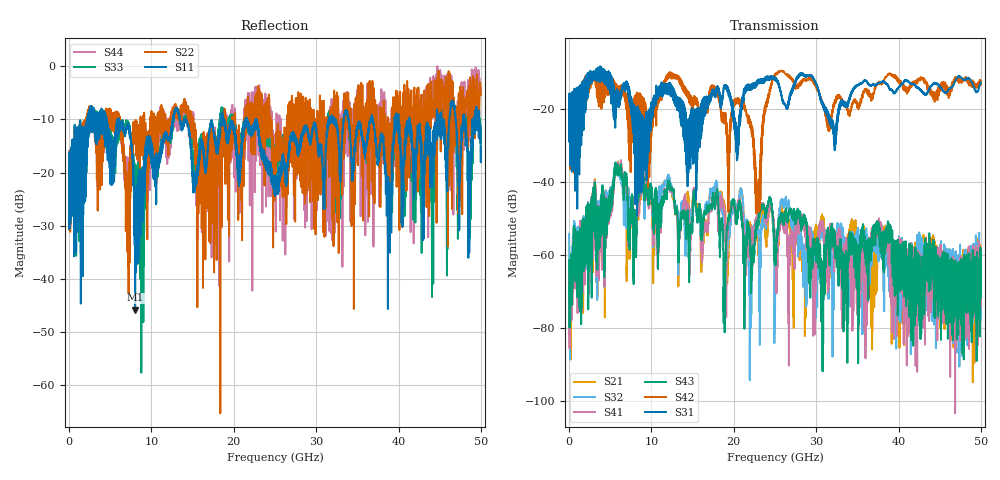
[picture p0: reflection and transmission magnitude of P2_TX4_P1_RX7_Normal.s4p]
!Keysight Technologies,N5225B,MY57041031,A.13.20.10
!Date: Friday, May 31, 2019 11:25:08
!Correction: S11(Full 4 Port(1,2,3,4))
!S12(Full 4 Port(1,2,3,4))
!S13(Full 4 Port(1,2,3,4))
!S14(Full 4 Port(1,2,3,4))
!S21(Full 4 Port(1,2,3,4))
!S22(Full 4 Port(1,2,3,4))
!S23(Full 4 Port(1,2,3,4))
!S24(Full 4 Port(1,2,3,4))
!S31(Full 4 Port(1,2,3,4))
!S32(Full 4 Port(1,2,3,4))
!S33(Full 4 Port(1,2,3,4))
!S34(Full 4 Port(1,2,3,4))
!S41(Full 4 Port(1,2,3,4))
!S42(Full 4 Port(1,2,3,4))
!S43(Full 4 Port(1,2,3,4))
!S44(Full 4 Port(1,2,3,4))
!S4P File: Measurements: <S11,S12,S13,S14>,
!<S21,S22,S23,S24>,
!<S31,S32,S33,S34>,
!<S41,S42,S43,S44>:
# Hz S  dB  R 50.0
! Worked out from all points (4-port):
!   5000 points, 10 MHz to 50 GHz, reference 50 ohm
!   strongest paths, dB at 10 MHz, 12.51 GHz, 25.01 GHz, 37.51 GHz, 50 GHz:
!     S31: -19.4, -14.3, -11.3, -12.8, -12.6
!     S42: -19.7, -10.0, -10.7, -12.7, -12.1
!     S43: -61.4, -41.9, -59.2, -51.4, -65.4
!     S41: -64.8, -42.2, -56.3, -50.8, -69.2
!     S32: -54.2, -42.4, -77.3, -54.0, -59.1
!     S21: -56.5, -43.2, -65.8, -56.1, -67.4
!   lowest |S11| = -45.8 dB at 8.03 GHz (marker M1), VSWR 1.01, Z = 50.2 - j0.469 ohm
!   |S11| at or under -10 dB: 6.073 GHz to 12.61 GHz (6.542 GHz wide, 70 % of centre); 14.21 GHz to 18.43 GHz (4.227 GHz wide, 25.9 % of centre); 22.71 GHz to 31.52 GHz (8.807 GHz wide, 32.5 % of centre)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
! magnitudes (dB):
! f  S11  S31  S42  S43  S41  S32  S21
! 10 MHz  -18.9  -19.4  -19.7  -61.4  -64.8  -54.2  -56.5
! 5.76 GHz  -13.2  -18.0  -16.5  -35.5  -35.5  -35.6  -35.4
! 8.03 GHz  -45.8  -23.3  -17.5  -51.9  -51.4  -52.3  -51.4
! 20.55 GHz  -18.0  -25.5  -16.9  -48.2  -47.2  -46.5  -45.9
! 22.93 GHz  -11.9  -12.4  -40.8  -51.8  -49.7  -51.9  -57.6
! 25.52 GHz  -19.0  -13.7  -9.7  -50.6  -53.3  -48.6  -52.3
! 50 GHz  -15.3  -12.6  -12.1  -65.4  -69.2  -59.1  -67.4
